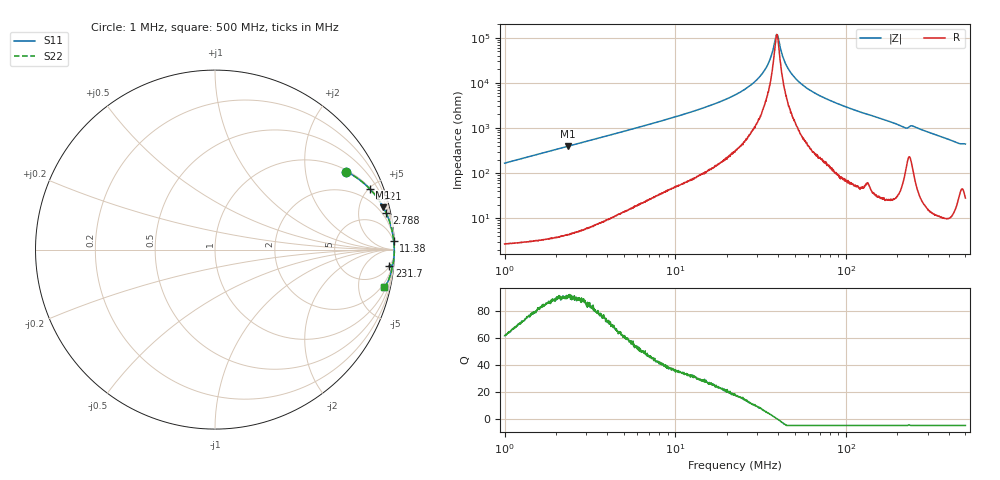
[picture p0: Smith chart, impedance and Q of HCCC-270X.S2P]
!s-Parameter Generated by FASTRON Sdn. Bhd.
!FASTRON P/N : HCCC-270X
!Keysight Technologies,E4991B,MY54100416,A.01.15
!Date: Mon Apr 06 16:09:43 2026
!Version  : Rev00 Mon Apr 06 16:09:43 2026
!Data & Calibration Information:
!PortZ  Port1:50+j0  Port2:50+j0
!When reading, reference impedance value at option line is always used.
!Remarks : This data is being provided solely for informational purposes.
!Freq	S11	S21	S12	S22
# Hz S dB R 50
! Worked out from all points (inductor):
!   1601 points, 1 MHz to 500 MHz, reference 50 ohm
!   read as one part in series: L = 26.5 uH near 1.032 MHz
!   highest Q = 90.7 at 2.35 MHz (marker M1), where L = 26.6 uH
!   self-resonance near 39.27 MHz
!   S11 on the Smith chart (normalised r, x): 1 MHz: 1.05, +3.33; 1.521 MHz: 1.06, +5.07; 2.788 MHz: 1.11, +9.33; 11.38 MHz: 2, +41; 231.7 MHz: 5, -20; 500 MHz: 1.56, -8.81
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1000000  -1.40 30.7  -5.83 -58.3  -5.83 -58.3  -1.40 30.7
1521180  -0.67 21.4  -8.75 -67.8  -8.75 -67.8  -0.67 21.4
2350219  -0.30 14.2  -12.18 -75.1  -12.18 -75.1  -0.30 14.2
2788239  -0.22 12.1  -13.59 -77.3  -13.59 -77.3  -0.22 12.1
2820919  -0.21 11.9  -13.69 -77.4  -13.69 -77.4  -0.21 11.9
7957584  -0.04 4.1  -22.81 -84.5  -22.81 -84.5  -0.04 4.1
1.137554e7  -0.02 2.8  -26.27 -85.5  -26.27 -85.5  -0.02 2.8
2.236068e7  -0.01 1.1  -34.67 -85.7  -34.67 -85.7  -0.01 1.1
2.790203e7  -0.01 0.6  -39.28 -84.2  -39.28 -84.2  -0.01 0.6
3.233973e7  -0.01 0.3  -44.21 -81.3  -44.21 -81.3  -0.01 0.3
3.536177e7  -0.01 0.2  -49.33 -75.2  -49.33 -75.2  -0.01 0.2
3.851633e7  -0.01 0.0  -59.38 -38.4  -59.38 -38.4  -0.01 0.0
3.942448e7  -0.01 -0.0  -61.11 3.0  -61.11 3.0  -0.01 -0.0
4.344476e7  -0.01 -0.2  -49.89 75.5  -49.89 75.5  -0.01 -0.2
4.677219e7  -0.01 -0.3  -45.23 81.1  -45.23 81.1  -0.01 -0.3
5.296233e7  -0.01 -0.5  -40.48 84.6  -40.48 84.6  -0.01 -0.5
6.307767e7  -0.01 -0.9  -36.22 86.4  -36.22 86.4  -0.01 -0.9
9.374216e7  -0.01 -1.8  -30.16 86.8  -30.16 86.8  -0.01 -1.8
1.77937e8  -0.03 -4.1  -23.01 84.9  -23.01 84.9  -0.03 -4.1
2.317248e8  -0.21 -5.3  -20.44 72.5  -20.44 72.5  -0.21 -5.3
2.465825e8  -0.12 -5.1  -20.95 78.9  -20.95 78.9  -0.12 -5.1
5e8  -0.33 -12.6  -13.23 73.8  -13.23 73.8  -0.33 -12.6
